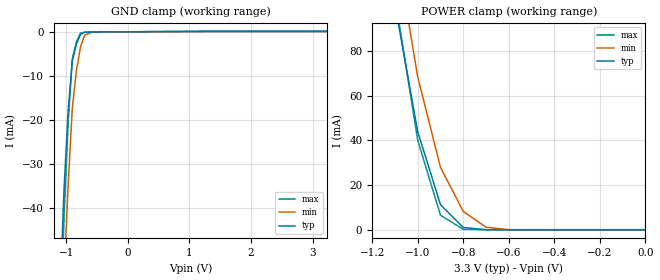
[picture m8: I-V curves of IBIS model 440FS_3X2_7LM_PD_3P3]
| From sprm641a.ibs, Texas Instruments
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|IQ0440FS_3X2_7LM_3P3; PULLDOWN_OFF
|   Model Cell 440FS_3X2_7LM_PD_3P3
|IQ0440FS_3X2_7LM_PD_3P3
[Model]   440FS_3X2_7LM_PD_3P3
Model_type   Input
Polarity   Non-Inverting
Vinl =  1.25
Vinh =  1.65
C_comp   1.2p   1.2p   1.2p
[Model Spec]
Vinl   1.25   1.12   1.38
Vinh   1.65   1.45   1.75
[Temperature Range]   25   155   -40
[Voltage Range]   3.3   2.97   3.63
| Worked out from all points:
|   GND clamp passes 1 mA (typ) near -0.78 V on its own axis
|   POWER clamp passes 1 mA (typ) near -0.78 V on its own axis
[POWER_clamp]
|   voltage   I(typ)   I(min)   I(max)
-3.3V     1.823A     2.351A     1.96A
-1.1V     100.7mA    129.7mA    104mA
-1.067V   81.79mA    109.2mA    82.71mA
-1.033V   62.86mA    88.78mA    61.4mA
-1V       43.93mA    68.32mA    40.09mA
-900mV    11.35mA    27.98mA    6.644mA
-800mV    1.193mA    8.315mA    343.1uA
-700mV    131.4uA    1.273mA    170.7uA
-600mV    97.55uA    154.6uA    168.7uA
0V        96.5uA     44.2uA     168.6uA
[GND_clamp]
|   voltage   I(typ)   I(min)   I(max)
-3.3V     -1.38A     -1.323A    -2.074A
-1.1V     -59.6mA    -79.12mA   -70.72mA
-1.033V   -35.49mA   -55.25mA   -41.83mA
-966.7mV  -17.83mA   -34.66mA   -20.31mA
-900mV    -6.6mA     -17.33mA   -6.147mA
-833.3mV  -2.744mA   -8.865mA   -2.295mA
-766.7mV  -575.7uA   -3.35mA    -279.2uA
-700mV    -96.31uA   -786.8uA   -98.86uA
-566.7mV  -52.15uA   -88.15uA   -76.87uA
3.233V    96.49uA    44.27uA    168.5uA
